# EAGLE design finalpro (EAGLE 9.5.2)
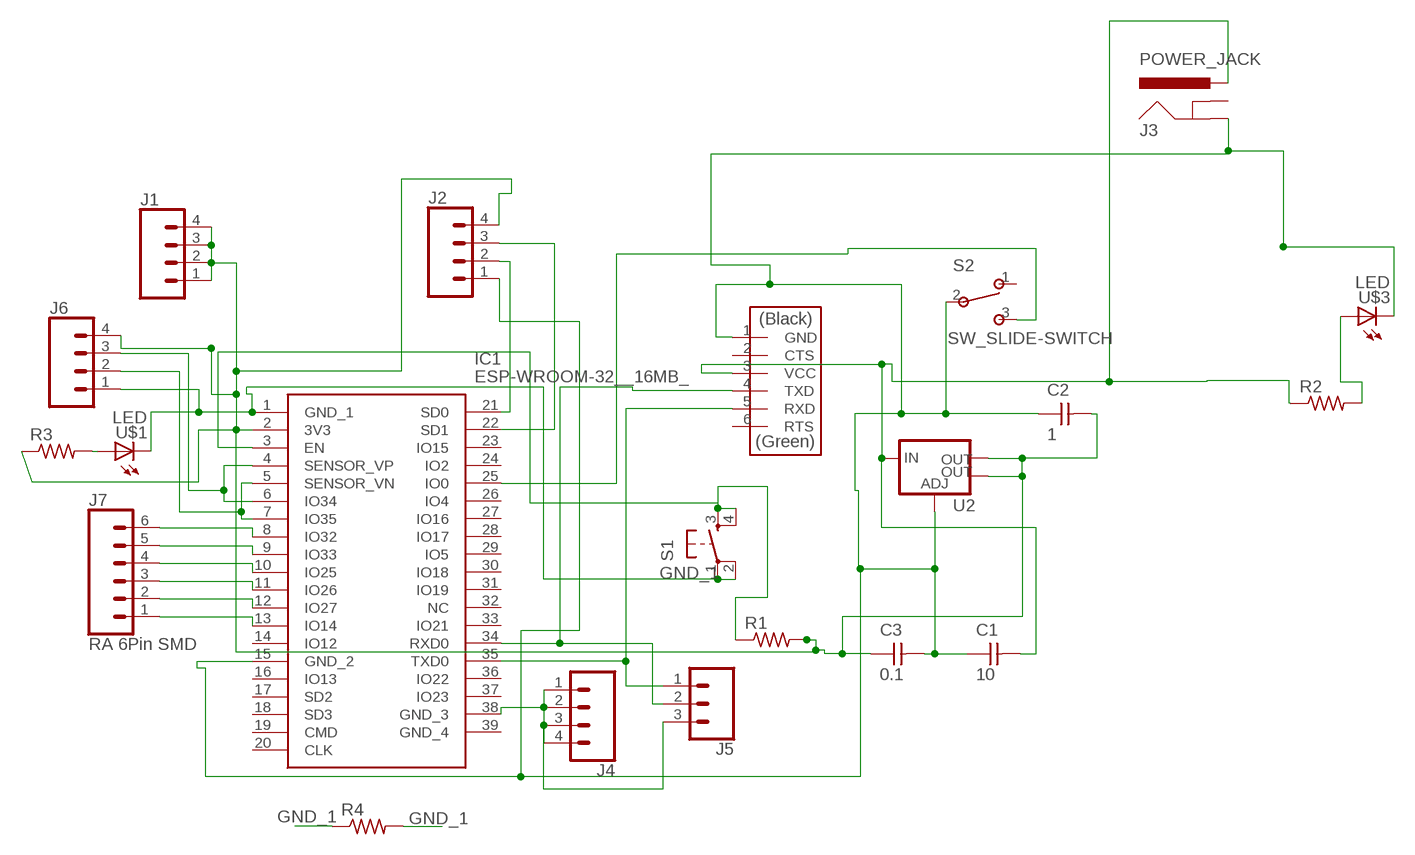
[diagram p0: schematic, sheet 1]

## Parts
C1  10  CAP_UNPOLARIZED  [C1206]
C2  1  CAP_UNPOLARIZED  [C1206]
C3  0.1  CAP_UNPOLARIZED  [C1206]
IC1  ESP-WROOM-32__16MB_  [ESP32WROOM32D]
J1  CONN_04LONGPADS  [1X04_LONGPADS]
J2  CONN_04LONGPADS  [1X04_LONGPADS]
J3  POWER_JACK  [POWER_JACK_PTH]
J4  CONN_04LONGPADS  [1X04_LONGPADS]
J5  CONN_03LONGPADS  [1X03_LONGPADS]
J6  CONN_04LONGPADS  [1X04_LONGPADS]
J7  RA 6Pin SMD  CONN_06SMD  [1X06-SMD_RA_MALE]
R1  R1206  [R1206]
R2  R1206  [R1206]
R3  R1206  [R1206]
R4  R1206  [R1206]
S1  SW_SWITCH_TACTILE_6MM6MM_SWITCH  [6MM_SWITCH]
S2  SW_SLIDE-SWITCH  [AYZ0102AGRLC]
U2  VR_REGULATOR_LM1117SOT223  [SOT223]
U$1  LED  [LED1206]
U$2  CONN_06_FTDI-SMD-HEADER  [1X06SMD]
U$3  LED  [LED1206]

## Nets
GND_1: IC1.1(GND_1) J6.1 R4.1 R4.2 S1.1(P) S1.2(P1) U$1.2(C)
N$2: IC1.3(EN) R1.1 S1.3(S) S1.4(S1)
N$3: IC1.25(IO0) S2.3
N$4: IC1.4(SENSOR_VP) IC1.6(IO34) J6.3
N$5: C1.2 J3.PWR R2.1 U2.3(IN) U$2.3(VCC)
N$6: IC1.38(GND_3) J4.1 J4.2 J4.3 J4.4 J5.3
N$8: IC1.35(TXD0) J5.1 U$2.5(RXD)
N$9: C2.2 C3.1 IC1.2(3V3) J1.1 J1.2 J1.3 J1.4 J2.4 J6.4 R1.2 R3.1 U2.2(OUT) U2.4(OUT)
N$10: C1.1 C2.1 C3.2 IC1.15(GND_2) J2.1 J3.GND S2.2 U2.1(ADJ) U$2.1(GND) U$3.2(C)
N$11: R2.2 U$3.1(A)
N$12: IC1.5(SENSOR_VN) IC1.7(IO35) J6.2
N$13: R3.2 U$1.1(A)
N$14: IC1.8(IO32) J7.6
N$15: IC1.21(SD0) J2.2
N$17: IC1.22(SD1) J2.3
N$18: IC1.9(IO33) J7.5
N$19: IC1.10(IO25) J7.4
N$20: IC1.11(IO26) J7.3
N$21: IC1.12(IO27) J7.2
N$22: IC1.13(IO14) J7.1
N$23: IC1.34(RXD0) J5.2 U$2.4(TXD)
Unconnected: IC1.14(IO12) IC1.16(IO13) IC1.17(SD2) IC1.18(SD3) IC1.19(CMD) IC1.20(CLK) IC1.23(IO15) IC1.24(IO2) IC1.26(IO4) IC1.27(IO16) IC1.28(IO17) IC1.29(IO5) IC1.30(IO18) IC1.31(IO19) IC1.32(NC) IC1.33(IO21) IC1.36(IO22) IC1.37(IO23) IC1.39(GND_4) J3.GNDBREAK S2.1 U$2.2(CTS) U$2.6(RTS)

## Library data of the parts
C1-C3 = eagle_fab:CAP_UNPOLARIZED
IC1 = ESP-WROOM-32__16MB_:ESP-WROOM-32__16MB_: WiFi Modules (802.11) SMD Module, ESP32-D0WDQ6, 128Mbits SPI flash, UART Mode Source: Datasheet; DESCRIPTION: WiFi Modules (802.11) SMD Module, ESP32-D0WDQ6, 128Mbits SPI flash, UART Mode; HEIGHT: 3.1mm; MANUFACTURER_NAME: Espressif; MANUFACTURER_PART_NUMBER: ESP-WROOM-32 (16MB); MOUSER_PART_NUMBER: 356-ESPWROOM3216MB
J1 J2 J4 J6 = SparkFun-Connectors:CONN_04: Multi connection point. Often used as Generic Header-pin footprint for 0.1 inch spaced/style header connections On any of the 0.1 inch spaced packages, you can populate with these: Break Away Headers - Straight (PRT-00116) Break Away Male Headers - Right Angle (PRT-00553) Female Headers (PRT-00115)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; PROD_ID: CONN-09696
J3 = SparkFun-Connectors:POWER_JACK: Power Jack Connector This is the standard 5.5mm barrel jack for power. The PTH is the most common, proven, reliable, footprint. The Slot footprint only works if the mill layer is transmitted to the PCB fab house so be warned. Here are the connectors we sell at SparkFun: DC Barrel Power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; PROD_ID: CONN-08197
J5 = SparkFun-Connectors:CONN_03: Multi connection point. Often used as Generic Header-pin footprint for 0.1 inch spaced/style header connections On any of the 0.1 inch spaced packages, you can populate with these: Break Away Headers - Straight (PRT-00116) Break Away Male Headers - Right Angle (PRT-00553) Female Headers (PRT-00115)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
J7 = SparkFun-Connectors:CONN_06: Multi connection point. Often used as Generic Header-pin footprint for 0.1 inch spaced/style header connections On any of the 0.1 inch spaced packages, you can populate with these: Break Away Headers - Straight (PRT-00116) Break Away Male Headers - Right Angle (PRT-00553) Female Headers (PRT-00115)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; PROD_ID: CONN-08971
R1-R4 = eagle_fab:R: Resistor (US Symbol)
S1 = eagle_fab:SW_SWITCH_TACTILE_6MM: OMRON SWITCH
S2 = eagle_fab:SW_SLIDE-SWITCH: SMD slide-switch AYZ0102AGRLC as found in the fablab inventory. Includes the mounting holes. Made by Zaerc.
U2 = eagle_fab:VR_REGULATOR_LM1117: Voltage Regulator LM1117 Standard adjustable voltage regulator but in SMD form. Spark Fun Electronics SKU : COM-00595; PROD_ID: VREG-08170
U$1 U$3 = eagle_fab:LED: LED
U$2 = eagle_fab:CONN_06_FTDI-SMD-HEADER

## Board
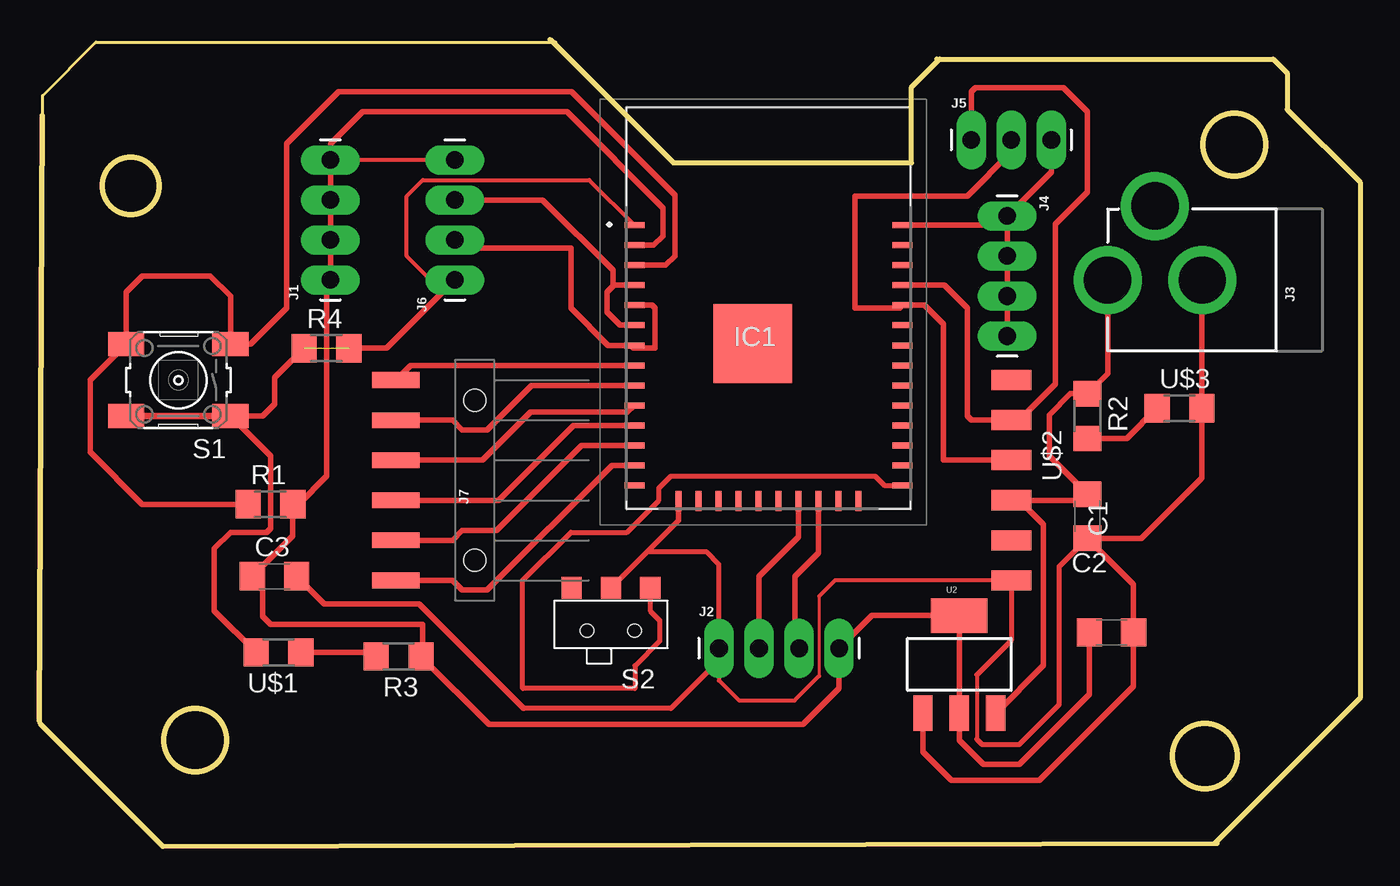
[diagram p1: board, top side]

Size 83.77 x 51.21 mm. Coordinates in mm from the lower left corner, seen from the top.
Outline: 0.18,46.36 0,8
Outline: 0.2,45.87 0.2,47.65 3.58,51.03 32.74,51.03
Outline: 56.92,49.96 57.1,49.96
Outline: 57.1,49.96 78.26,49.96 79.15,49.07 79.15,46.76 83.77,42.14 83.77,9.42 74.52,0.18
Outline: 74.7,0.18 7.85,0 0.03,7.82
Outline: 32.38,51.21 40.21,43.38 55.32,43.38 55.32,48.18 57.1,49.96
Outline: circle at 5.79,41.91 radius 1.8
Outline: circle at 9.88,6.76 radius 1.98
Outline: circle at 75.79,44.53 radius 1.98
Outline: circle at 73.91,5.74 radius 2.05
Copper layers (1*16): Top 0.035mm / dielectric 1.5mm / Bottom 0.035mm
Design rules "default *": minimum track width 6mil, minimum drill 0.35mm, track to track 16mil, track to pad 6mil, pad to pad 6mil, via to via 6mil, smd to smd 6mil, copper to edge 40mil, drill to drill 6mil, minimum pad ring 10mil, minimum via ring 8mil, stop-mask expansion 4mil, vias tented up to drill 0mil, thermal gap 10mil

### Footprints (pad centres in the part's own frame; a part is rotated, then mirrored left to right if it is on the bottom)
C1206 = smd 1.6 x 1.8: 1 -1.4,0; 2 1.4,0
ESP32WROOM32D = smd 1.27 x 0.381: 1 -8.15,5.51; 2 -8.15,4.24; 3 -8.15,2.97; 4 -8.15,1.7; 5 -8.15,0.43; 6 -8.15,-0.84; 7 -8.15,-2.11; 8 -8.15,-3.38; 9 -8.15,-4.65; 10 -8.15,-5.92; 11 -8.15,-7.19; 12 -8.15,-8.46; 13 -8.15,-9.73; 14 -8.15,-11; 25 8.85,-11; 26 8.85,-9.73; 27 8.85,-8.46; 28 8.85,-7.19; 29 8.85,-5.92; 30 8.85,-4.65; 31 8.85,-3.38; 32 8.85,-2.11; 33 8.85,-0.84; 34 8.85,0.43; 35 8.85,1.7; 36 8.85,2.97; 37 8.85,4.24; 38 8.85,5.51 | smd 0.381 x 1.27: 15 -5.365,-12; 16 -4.095,-12; 17 -2.825,-12; 18 -1.555,-12; 19 -0.285,-12; 20 0.985,-12; 21 2.255,-12; 22 3.525,-12; 23 4.795,-12; 24 6.065,-12 | smd 5 x 5: 39 -0.65,-1.99
1X04_LONGPADS = drill 1.118 pad 1.88 long: 1 0,0; 2 2.54,0; 3 5.08,0; 4 7.62,0
POWER_JACK_PTH = drill 2.997 pad 4.318: GND 0,7.7; GNDBREAK 4.7,10.7; PWR 0,13.7
1X03_LONGPADS = drill 1.118 pad 1.88 long: 1 0,0; 2 2.54,0; 3 5.08,0
1X06-SMD_RA_MALE = smd 1 x 3: 1 -6.35,5; 2 -3.81,5; 3 -1.27,5; 4 1.27,5; 5 3.81,5; 6 6.35,5 | hole 1.4: -5.08,0; 5.08,0
R1206 = smd 1.6 x 1.803: 1 -1.422,0; 2 1.422,0
6MM_SWITCH = smd 2.286 x 1.524: 1 -3.302,2.286; 2 3.302,2.286; 3 -3.302,-2.286; 4 3.302,-2.286
AYZ0102AGRLC = smd 1.27 x 1.397: 1 2.5,-2.3; 2 0,-2.3; 3 -2.5,-2.3 | hole 0.85: -1.5,0.4; 1.5,0.4
SOT223 = smd 1.219 x 2.235: 1 -2.311,-3.099; 2 0,-3.099; 3 2.311,-3.099 | smd 3.6 x 2.2: 4 0,3.099
LED1206 = smd 1.6 x 1.803: 1 -1.422,0; 2 1.422,0
1X06SMD = smd 2.54 x 1.27: 1 0,6.35; 2 0,3.81; 3 0,1.27; 4 0,-1.27; 5 0,-3.81; 6 0,-6.35

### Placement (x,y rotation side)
C1  66.47,20.95 90 top
C2  68,13.59 180 top
C3  14.91,17.14 0 top
IC1  45.9,33.91 0 top
J1  18.47,35.94 90 top
J2  43.1,12.57 0 top
J3  81.46,35.94 90 top
J4  61.39,40 270 top
J5  59.11,44.83 0 top
J6  26.34,35.94 90 top
J7  27.61,23.24 90 top
R1  14.66,21.72 0 top
R2  66.47,27.3 270 top
R3  22.78,12.06 180 top
R4  18.21,31.62 0 top
S1  8.81,29.59 180 top
S2  36.25,14.1 180 top
U2  58.34,11.56 0 top
U$1  15.16,12.32 180 top
U$2  61.65,23.24 180 top
U$3  72.31,27.81 0 top

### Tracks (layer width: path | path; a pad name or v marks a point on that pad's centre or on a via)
GND_1  (1 unrouted)
  Top 0.254: J6.1 24.82,35.94 23.29,37.47 23.29,41.27 24.31,42.29 34.88,42.29 IC1.1
  Top 0.356: R4.1 14.91,29.74 14.91,28.07 14.15,27.3 S1.1 14.66,24.77 14.66,20.19 14.4,19.94 12.12,19.94 11.1,18.92 11.1,14.96 U$1.2 | R4.2 22.02,31.62 J6.1
  Top 0.406: S1.2 S1.1
N$2
  Top 0.356: R1.1 6.53,21.72 3.23,25.02 3.23,29.59 S1.4 5.51,35.18 6.53,36.19 10.85,36.19 12.12,34.92 S1.3 13.39,31.88 15.67,34.16 15.67,44.58 18.97,47.88 33.77,47.88 40.31,41.34 40.31,37.47 39.72,36.88 IC1.3
N$3
  Top 0.305: S2.3 38.75,14.95 39.34,14.36 39.34,13.04 37.77,11.47 37.77,10.03 30.66,10.03 30.66,16.89 33.71,19.94 37.26,19.94 39.29,21.97 39.29,22.73 40.06,23.49 53.01,23.49 53.6,22.91 IC1.25
N$4
  Top 0.356: IC1.4 36.42,35.61 36.37,35.56 | 36.37,35.56 35.99,35.18 35.99,33.91 36.83,33.07 IC1.6 | J6.3 31.93,41.02 36.37,36.58 36.37,35.56
N$5
  Top 0.356: J3.PWR 67.76,30.01 R2.1 65.4,28.73 64.06,27.38 64.06,24.77 C1.2 66.09,21.97 U$2.3 62.15,21.97 63.68,20.45 63.68,11.48 U2.3
N$6
  Top 0.356: J5.3 64.19,42.8 J4.1 | J4.1 60.81,39.42 IC1.38 | J4.1 J4.2 J4.3 J4.4
N$8
  Top 0.356: IC1.35 57.41,35.61 58.85,34.16 58.85,27.3 59.11,27.05 U$2.5 62.15,27.05 64.44,29.34 64.44,39.5 66.47,41.53 66.47,46.61 64.95,48.13 59.36,48.13 59.11,47.88 J5.1
N$9
  Top 0.254: J6.4 J1.4
  Top 0.356: IC1.2 38.96,38.15 39.55,38.73 39.55,40.51 33.45,46.61 20.5,46.61 18.47,44.58 J1.4 J1.3 J1.2 J1.1 18.21,35.69 18.21,23.49 16.43,21.72 R1.2 16.08,19.71 C3.1 14.15,16.51 14.15,14.61 14.66,14.1 24.31,14.1 24.31,12.06 24.26,12.01 | C2.2 66.6,9.65 62.15,5.21 59.87,5.21 58.34,6.73 U2.2 U2.4 52.81,14.66 J2.4 50.72,10.03 48.44,7.75 28.52,7.75 24.26,12.01 | R3.1 24.26,12.01
N$10
  Top 0.203: 49.45,15.88 49.45,10.82
  Top 0.254: J2.1 43.1,10.54 44.37,9.27 47.9,9.27 49.45,10.82 | U$2.1 50.47,16.89 49.45,15.88 | 59.46,10.9 59.46,6.81
  Top 0.305: U$2.1 61.65,13.08 59.46,10.9 | 59.46,6.81 59.79,6.48 62.15,6.48 64.69,9.02 64.69,17.78 C1.1 | S2.2 38.52,18.68 | 38.52,18.68 40.53,20.68 | 38.52,18.68 42.33,18.68 43.1,17.91 J2.1 43.1,11.81 40.06,8.76 30.72,8.76
  Top 0.356: J3.GND 73.74,35.92 U$3.2 73.74,23.39 69.9,19.55 C1.1 69.4,16.63 C2.1 69.4,10.16 63.42,4.19 57.84,4.19 56.03,5.99 U2.1 | C3.2 18.06,15.39 24.09,15.39 30.72,8.76 | 40.53,20.68 IC1.15
N$11
  Top 0.356: R2.2 68.96,25.88 U$3.1
N$12
  Top 0.356: IC1.5 38.86,34.34 39.04,34.16 39.04,31.62 37.69,31.62 37.52,31.8 | J6.2 26.85,37.97 33.71,37.97 33.71,34.16 36.07,31.8 37.52,31.8 | 37.52,31.8 IC1.7
N$13
  Top 0.356: U$1.1 21.11,12.32 R3.2
N$14
  Top 0.356: IC1.8 23.55,30.53 J7.6
N$15
  Top 0.356: IC1.21 48.15,19.65 45.64,17.14 J2.2
N$17
  Top 0.356: IC1.22 49.42,18.64 47.93,17.14 47.93,12.83 J2.3
N$18
  Top 0.356: IC1.9 31.23,29.26 28.39,26.43 26.83,26.43 26.2,27.05 J7.5
N$19
  Top 0.356: IC1.10 37.32,27.56 31.17,27.56 28.12,24.51 J7.4
N$20
  Top 0.356: IC1.11 33.88,26.72 29.13,21.97 J7.3
N$21
  Top 0.356: IC1.12 34.39,25.45 29,20.05 26.83,20.05 26.2,19.43 J7.2
N$22
  Top 0.356: IC1.13 36.31,24.18 28.39,16.27 26.83,16.27 26.2,16.89 J7.1
N$23
  Top 0.356: J5.2 61.65,44.07 58.85,41.27 51.74,41.27 51.74,34.16 54.57,34.16 IC1.34 56.14,34.34 57.33,33.15 57.33,24.51 U$2.4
